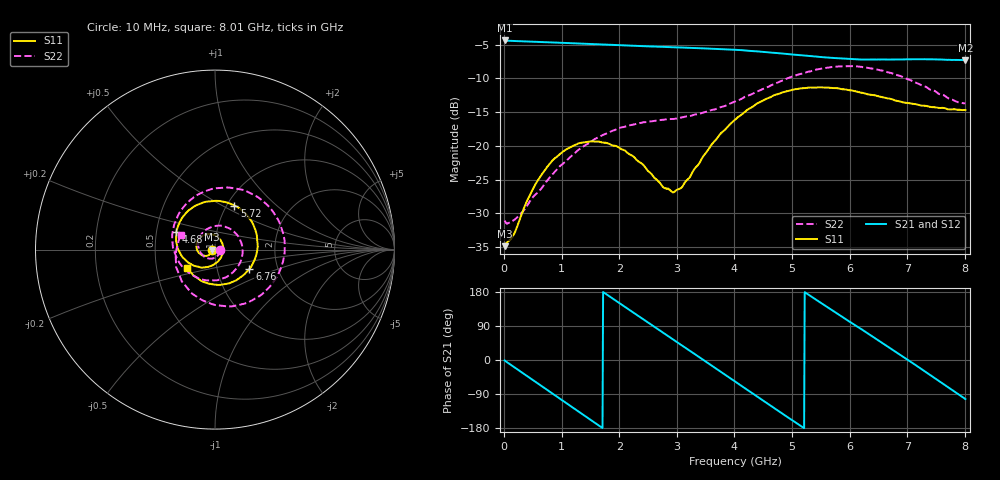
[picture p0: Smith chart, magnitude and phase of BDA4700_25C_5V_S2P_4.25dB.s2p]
!Agilent Technologies,E5071B,MY42404982,A.09.10
!Date: Mon Oct 20 13:28:01 2025
!Data & Calibration Information:
!Freq	S11:SOLT2(ON)	S21:SOLT2(ON)	S12:SOLT2(ON)	S22:SOLT2(ON)
# Hz S RI R 50
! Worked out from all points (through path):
!   801 points, 10 MHz to 8.01 GHz, reference 50 ohm
!   highest |S21| = -4.37 dB at 10 MHz (marker M1); lowest = -7.3 dB at 8.01 GHz (marker M2)
!   group delay of S21, straight-line fit = 284 ps
!   lowest |S11| = -34.8 dB at 10 MHz (marker M3), VSWR 1.04, Z = 48.2 - j0.121 ohm
!   |S11| at or under -10 dB: start of sweep to end of sweep
!   |S22| runs from -31.5 to -8.2 dB; largest |S21 - S12| = 0.0048
!   S11 on the Smith chart (normalised r, x): 10 MHz: 0.96, -0.00; 4.68 GHz: 0.64, +0.13; 5.72 GHz: 1.09, +0.57; 6.76 GHz: 1.43, -0.32; 8.01 GHz: 0.72, -0.15
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1e7  -0.0181 -0.00126  0.6044 -0.0132  0.6045 -0.0136  0.028 -0.00253
3.3e8  -0.025 -0.0219  0.4861 -0.3439  0.4853 -0.3446  0.0202 -0.0259
7.2e8  -0.0572 -0.0353  0.1386 -0.5704  0.1385 -0.5706  -0.0181 -0.0503
1.02e9  -0.0884 -0.0196  -0.1767 -0.5526  -0.1773 -0.553  -0.0645 -0.0356
1.35e9  -0.1037 0.0202  -0.452 -0.3515  -0.4524 -0.3516  -0.0936 0.0263
1.93e9  -0.0544 0.0842  -0.5168 0.2123  -0.5167 0.2128  0.00286 0.1317
2.32e9  0.00276 0.0774  -0.2535 0.4876  -0.2534 0.488  0.1137 0.0925
2.68e9  0.0398 0.0373  0.0897 0.5361  0.0896 0.5358  0.1536 -0.0192
2.96e9  0.0447 -0.00918  0.3332 0.4219  0.3335 0.4215  0.1171 -0.1072
3.36e9  0.0104 -0.0708  0.5215 0.0969  0.5223 0.0964  -0.00401 -0.1718
3.67e9  -0.0503 -0.098  0.4871 -0.1914  0.4869 -0.1925  -0.1125 -0.1496
4.01e9  -0.1327 -0.0821  0.2831 -0.4304  0.2834 -0.43  -0.2031 -0.0654
4.34e9  -0.1984 -0.0124  -0.00689 -0.5035  -0.00697 -0.5042  -0.238 0.0636
4.68e9  -0.2151 0.0992  -0.287 -0.3965  -0.2871 -0.3977  -0.1951 0.2105
5.02e9  -0.1568 0.2095  -0.4482 -0.1574  -0.4495 -0.1575  -0.0634 0.3225
5.35e9  -0.0415 0.2676  -0.4483 0.1125  -0.4485 0.1117  0.1211 0.339
5.72e9  0.1084 0.2455  -0.2821 0.3489  -0.2815 0.3494  0.3105 0.2279
6.18e9  0.2261 0.1045  0.0492 0.4343  0.052 0.4351  0.3833 -0.046
6.68e9  0.2082 -0.0842  0.3628 0.2424  0.364 0.2418  0.2062 -0.2832
6.76e9  0.1915 -0.108  0.3932 0.1897  0.3942 0.1878  0.1632 -0.3015
7.3e9  0.0282 -0.1966  0.3825 -0.215  0.3822 -0.2158  -0.1245 -0.2475
8.01e9  -0.1555 -0.0998  -0.0982 -0.4203  -0.0981 -0.421  -0.1895 0.0825
